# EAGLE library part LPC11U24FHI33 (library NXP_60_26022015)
32-bit ARM Cortex-M0 microcontroller; up to 32 kB flash; up to 10 kB SRAM and 4 kB EEPROM; USB device; USART The LPC11U2x are an ARM Cortex-M0 based, low-cost 32-bit MCU family, designed for 8/16-bit microcontroller applications, offering performance, low power, simple instruction set and memory addressing together with reduced code size compared to existing 8/16-bit architectures. The LPC11U2x operate at CPU frequencies of up to 50 MHz. Equipped with a highly flexible and configurable Full-Speed USB 2.0 device controller, the LPC11U2x brings unparalleled design flexibility and seamless integration to today’s demanding connectivity solutions. The peripheral complement of the LPC11U2x includes up to 32 kB of flash memory, up to 10 kB of SRAM data memory and 4 kB EEPROM, one Fast-mode Plus I 2 C-bus interface, one RS-485/EIA-485 USART with support for synchronous mode and smart card interface, two SSP interfaces, four general-purpose counter/timers, a 10-bit ADC (Analog-to-Digital Converter), and up to 54 general-purpose I/O pins. AAL Eindhoven MK
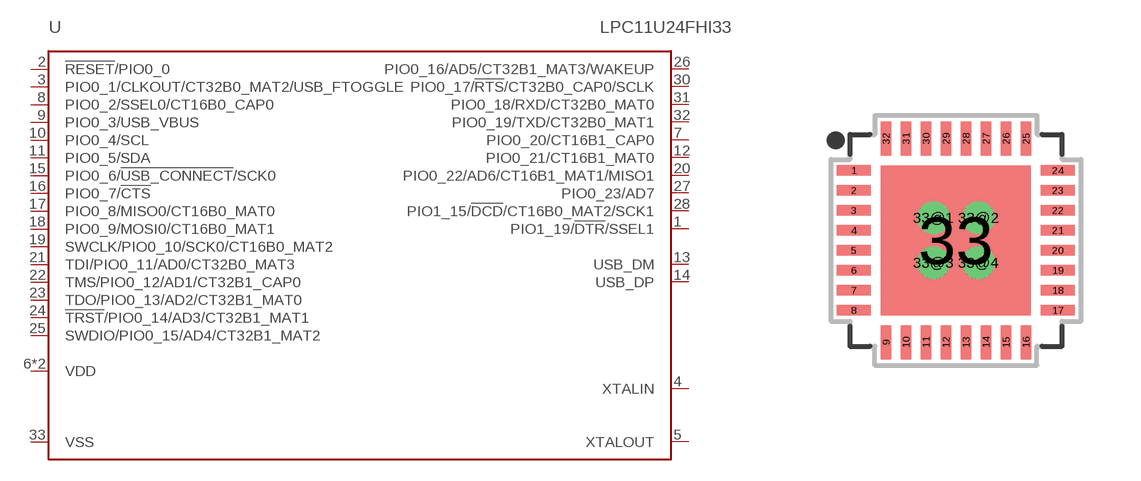
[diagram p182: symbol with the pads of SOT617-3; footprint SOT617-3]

Designator prefix U

## LPC11U24FHI33/301 (EEPROM: 2kB; FLASH: 32kB; GPIO: 26; SRAM: 6kB; USB_SRAM: 2kB)  [SOT617-3]
1  PIO1_19/!DTR!/SSEL1
2  !RESET!/PIO0_0
3  PIO0_1/CLKOUT/CT32B0_MAT2/USB_FTOGGLE
4  XTALIN  in
5  XTALOUT  out
6  VDD  pwr
7  PIO0_20/CT16B1_CAP0
8  PIO0_2/SSEL0/CT16B0_CAP0
9  PIO0_3/USB_VBUS
10  PIO0_4/SCL
11  PIO0_5/SDA
12  PIO0_21/CT16B1_MAT0
13  USB_DM
14  USB_DP
15  PIO0_6/!USB_CONNECT!/SCK0
16  PIO0_7/!CTS!
17  PIO0_8/MISO0/CT16B0_MAT0
18  PIO0_9/MOSI0/CT16B0_MAT1
19  SWCLK/PIO0_10/SCK0/CT16B0_MAT2
20  PIO0_22/AD6/CT16B1_MAT1/MISO1
21  TDI/PIO0_11/AD0/CT32B0_MAT3
22  TMS/PIO0_12/AD1/CT32B1_CAP0
23  TDO/PIO0_13/AD2/CT32B1_MAT0
24  !TRST!/PIO0_14/AD3/CT32B1_MAT1
25  SWDIO/PIO0_15/AD4/CT32B1_MAT2
26  PIO0_16/AD5/CT32B1_MAT3/WAKEUP
27  PIO0_23/AD7
28  PIO1_15/!DCD!/CT16B0_MAT2/SCK1
29  VDD  pwr
30  PIO0_17/!RTS!/CT32B0_CAP0/SCLK
31  PIO0_18/RXD/CT32B0_MAT0
32  PIO0_19/TXD/CT32B0_MAT1
33  VSS  pwr

## Footprint SOT617-3 (pad centres in mm)
SOT617-3 HVQFN32: plastic thermal enhanced very thin quad flat package; no leads; 32 terminals; body 5 x 5 x 0.85 mm JEDEC: MO-220 IEC: -- JEITA: --
smd 0.85 x 0.27: 1 -2.55,1.75; 2 -2.55,1.25; 3 -2.55,0.75; 4 -2.55,0.25; 5 -2.55,-0.25; 6 -2.55,-0.75; 7 -2.55,-1.25; 8 -2.55,-1.75; 17 2.55,-1.75; 18 2.55,-1.25; 19 2.55,-0.75; 20 2.55,-0.25; 21 2.55,0.25; 22 2.55,0.75; 23 2.55,1.25; 24 2.55,1.75
smd 0.27 x 0.85: 9 -1.75,-2.55; 10 -1.25,-2.55; 11 -0.75,-2.55; 12 -0.25,-2.55; 13 0.25,-2.55; 14 0.75,-2.55; 15 1.25,-2.55; 16 1.75,-2.55; 25 1.75,2.55; 26 1.25,2.55; 27 0.75,2.55; 28 0.25,2.55; 29 -0.25,2.55; 30 -0.75,2.55; 31 -1.25,2.55; 32 -1.75,2.55
smd 3.75 x 3.75: 33 0,0
drill 0.3 pad 0.6: 33@1 -0.562,0.562; 33@2 0.562,0.562; 33@3 -0.562,-0.562; 33@4 0.562,-0.562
